PROGRAM MAIN_FAST
(* This is the fast task and must run at the same rate as the NCI SAF Task *)
VAR
	iAxis			: USINT;	(* counter for the axis number *)
END_VAR

(* --------------------------------------------- *)
(* Triamec Motion AG, 6340 Baar, Switzerland     *)
(* Sample Code may be adapted to customer need   *)
(* --------------------------------------------- *)

(* Sync the trialink *)
gTrialink.CallFast();

FOR iAxis := 1 TO N_AXES DO
	(* get the coordinates from the NC and write it to the drive *)
	gAxes[iAxis].fastPositionCmd := gNciAxes[iAxis].CallFastPosCmd();
	gAxes[iAxis].CallFast(Trialink := gTrialink);

	(* get the actual position from the drive and pass it to NC *)
	gNciAxes[iAxis].CallFastPosAct(gAxes[iAxis].ActualPositionFast(Trialink := gTrialink));
END_FOR

publish1.CallFast(Trialink := gTrialink);

END_PROGRAM
